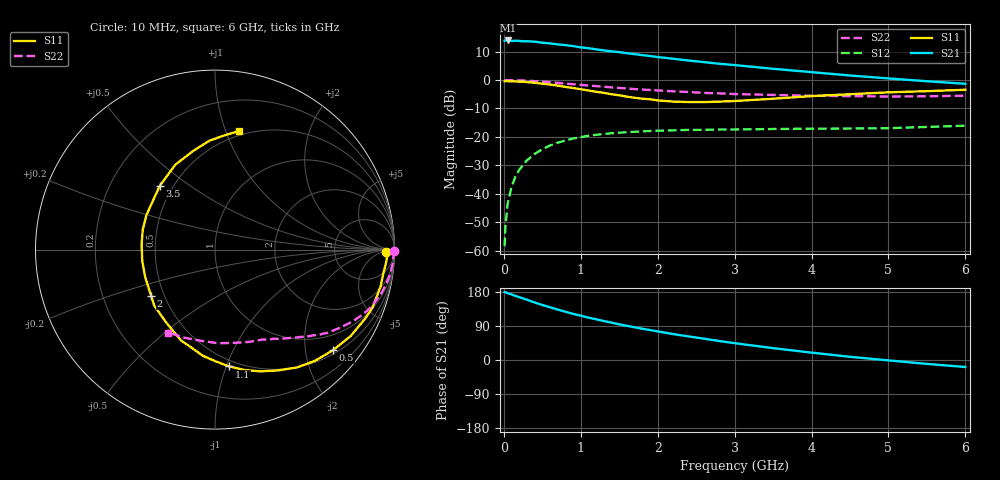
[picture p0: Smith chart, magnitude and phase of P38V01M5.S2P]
! SIEMENS Small Signal Semiconductors
! BFP181
! Si NPN RF Bipolar Junction Transistor in SOT143
! VCE = 8 V  IC = 1.5 mA
! Common Emitter S-Parameters:  March  1996
# GHz  S  MA  R  50
!  f  S11  S21  S12  S22
! GHz  MAG  ANG  MAG  ANG  MAG  ANG  MAG  ANG
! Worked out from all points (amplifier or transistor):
!   36 points, 10 MHz to 6 GHz, reference 50 ohm
!   highest |S21| = 13.9 dB at 50 MHz (marker M1)
!   |S21| within 3 dB of that: start of sweep to 1.168 GHz
!   unconditionally stable (mu >= 1): 2.856 GHz to end of sweep
!   at 250 MHz: K = 0.10, MSG = 21.8 dB, |S12| = -29.9 dB
!   at 1.4 GHz: K = 0.55, MSG = 14.4 dB, |S12| = -18.7 dB
!   at 6 GHz: K = 1.19, MAG = 4.7 dB, |S12| = -16.0 dB
!   S11 on the Smith chart (normalised r, x): 10 MHz: 38, -13; 500 MHz: 0.59, -2.60; 1.1 GHz: 0.45, -1.02; 2 GHz: 0.42, -0.27; 3.5 GHz: 0.42, +0.39; 6 GHz: 0.46, +1.12
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0.01  0.954 -0.9  4.921 179.3  0.0012 70.2  0.9965 -0.3
0.02  0.9596 -1.9  4.969 178.9  0.0026 97.3  0.9949 -0.7
0.05  0.957 -4.0  4.97 176.3  0.0068 89.7  0.9942 -2.0
0.1  0.9469 -8.2  4.854 173.0  0.0132 83.0  0.9954 -3.9
0.15  0.9452 -12.5  4.916 169.3  0.02 82.0  0.9899 -5.8
0.2  0.9385 -16.1  4.874 165.8  0.0264 79.7  0.9858 -7.7
0.3  0.9208 -24.7  4.821 159.3  0.0387 74.5  0.9728 -11.4
0.4  0.8962 -32.5  4.728 151.7  0.0502 69.4  0.9565 -15.1
0.5  0.864 -40.4  4.535 145.2  0.0607 64.2  0.9364 -18.4
0.6  0.8337 -48.0  4.413 139.1  0.0708 60.2  0.9164 -21.6
0.8  0.7589 -62.5  4.121 127.3  0.0865 52.1  0.8688 -27.1
0.9  0.7242 -69.5  3.955 121.8  0.0938 48.3  0.8439 -29.6
1.1  0.6556 -83.1  3.633 111.8  0.1049 42.0  0.8017 -34.0
1.5  0.5402 -110.6  3.103 94.1  0.1186 32.2  0.7263 -41.1
1.8  0.4704 -130.8  2.746 82.4  0.1254 27.0  0.6809 -45.6
2  0.4389 -144.1  2.539 75.5  0.1287 23.8  0.6572 -48.3
2.2  0.4186 -158.1  2.37 68.4  0.1303 21.0  0.6339 -51.2
2.8  0.4175 164.6  1.935 50.1  0.1351 14.9  0.5842 -59.3
3.5  0.4697 131.0  1.578 31.3  0.1379 10.5  0.5481 -69.7
4.5  0.5638 102.3  1.203 8.4  0.1406 6.4  0.5219 -88.3
5.5  0.6383 85.3  0.954 -10.3  0.1498 6.5  0.5194 -108.9
6  0.6758 78.4  0.859 -18.5  0.1576 5.5  0.5312 -119.6
